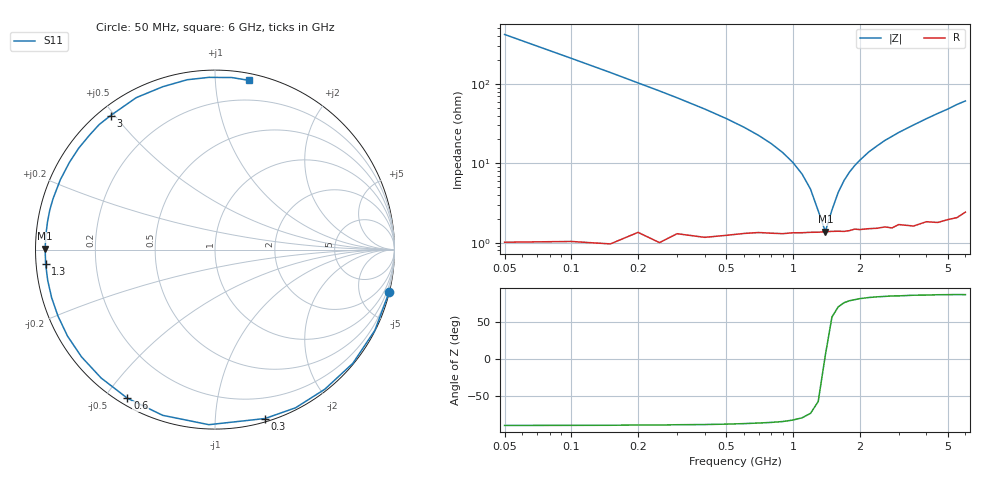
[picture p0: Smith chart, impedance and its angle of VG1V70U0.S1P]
! Infineon Technologies  Discrete & RF Semiconductors
! BB 831
! Si Tuning Diode in SOD323
! VR = 1.75 V
! S-Parameters:  July  1999
# GHz  S  MA  R  50
!  f  S11
! GHz  MAG  ANG
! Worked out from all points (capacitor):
!   34 points, 50 MHz to 6 GHz, reference 50 ohm
!   read as one part to ground: C = 7.54 pF near 50 MHz
!   lowest |Z| = 1.38 ohm at 1.4 GHz (marker M1)
!   series resonance near 1.394 GHz, so ESL is about 1.7 nH
!   S11 on the Smith chart (normalised r, x): 50 MHz: 0.02, -8.39; 300 MHz: 0.03, -1.34; 600 MHz: 0.03, -0.57; 1.3 GHz: 0.03, -0.04; 3 GHz: 0.03, +0.49; 6 GHz: 0.05, +1.22
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0.05  0.9994 -13.6
0.1  0.9978 -26.8
0.15  0.9956 -39.5
0.2  0.9897 -51.8
0.25  0.9891 -63.0
0.3  0.9815 -73.5
0.4  0.976 -92.0
0.5  0.9682 -107.5
0.6  0.9613 -120.5
0.7  0.9562 -131.6
0.8  0.9541 -141.2
0.9  0.9526 -149.6
1  0.9499 -157.0
1.1  0.9489 -163.6
1.3  0.9472 -175.1
1.4  0.9465 179.7
1.6  0.9459 170.7
1.8  0.9459 162.6
2  0.9455 155.6
2.4  0.9466 143.3
2.6  0.9464 137.6
3  0.9466 127.9
3.5  0.9536 117.4
4  0.953 107.8
4.5  0.959 99.3
5  0.9602 92.0
5.5  0.9632 84.4
6  0.9617 78.6
